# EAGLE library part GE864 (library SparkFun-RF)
Telit quad cell module (see CEL-09296)
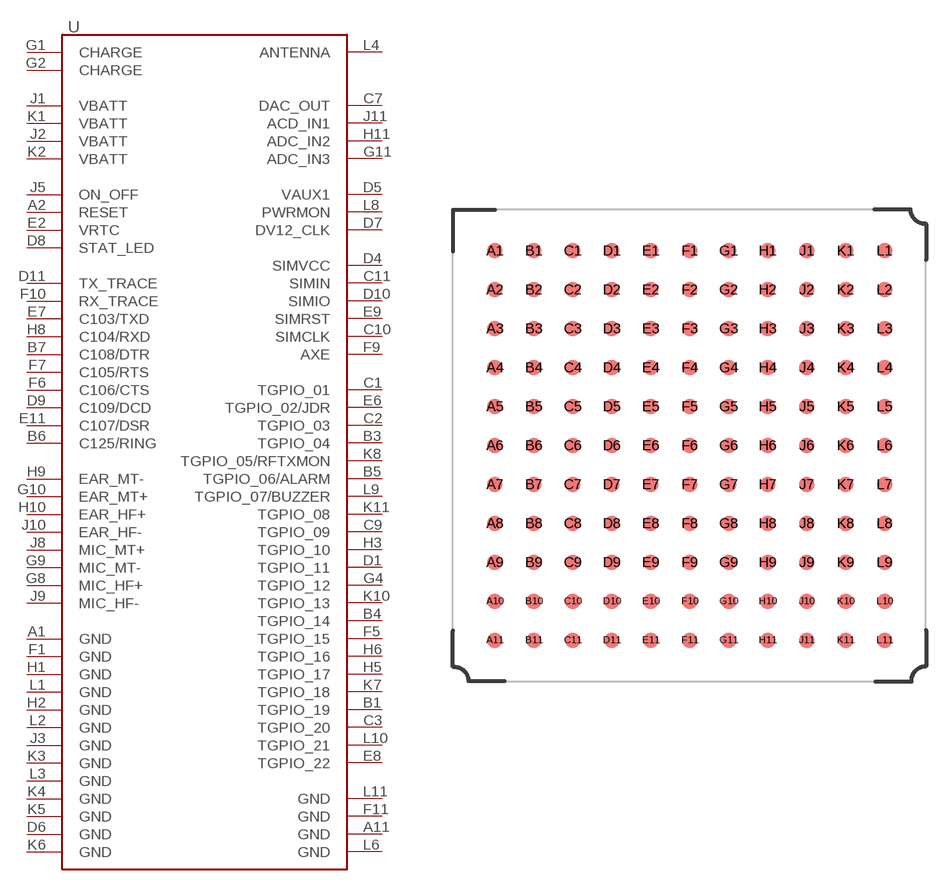
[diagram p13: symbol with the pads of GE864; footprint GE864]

Designator prefix -

## GE864  [GE864]
A1  GND
A2  RESET
A11  GND
B1  TGPIO_19
B3  TGPIO_04
B4  TGPIO_14
B5  TGPIO_06/ALARM
B6  C125/RING
B7  C108/DTR
C1  TGPIO_01
C2  TGPIO_03
C3  TGPIO_20
C7  DAC_OUT
C9  TGPIO_09
C10  SIMCLK
C11  SIMIN
D1  TGPIO_11
D4  SIMVCC
D5  VAUX1
D6  GND
D7  DV12_CLK
D8  STAT_LED
D9  C109/DCD
D10  SIMIO
D11  TX_TRACE
E2  VRTC
E6  TGPIO_02/JDR
E7  C103/TXD
E8  TGPIO_22
E9  SIMRST
E11  C107/DSR
F1  GND
F5  TGPIO_15
F6  C106/CTS
F7  C105/RTS
F9  AXE
F10  RX_TRACE
F11  GND
G1  CHARGE
G2  CHARGE
G4  TGPIO_12
G8  MIC_HF+
G9  MIC_MT-
G10  EAR_MT+
G11  ADC_IN3
H1  GND
H2  GND
H3  TGPIO_10
H5  TGPIO_17
H6  TGPIO_16
H8  C104/RXD
H9  EAR_MT-
H10  EAR_HF+
H11  ADC_IN2
J1  VBATT
J2  VBATT
J3  GND
J5  ON_OFF
J8  MIC_MT+
J9  MIC_HF-
J10  EAR_HF-
J11  ACD_IN1
K1  VBATT
K2  VBATT
K3  GND
K4  GND
K5  GND
K6  GND
K7  TGPIO_18
K8  TGPIO_05/RFTXMON
K10  TGPIO_13
K11  TGPIO_08
L1  GND
L2  GND
L3  GND
L4  ANTENNA
L6  GND
L8  PWRMON
L9  TGPIO_07/BUZZER
L10  TGPIO_21
L11  GND

## Footprint GE864 (pad centres in mm)
smd 1 x 1: A1 0,25; A2 0,22.5; A3 0,20; A4 0,17.5; A5 0,15; A6 0,12.5; A7 0,10; A8 0,7.5; A9 0,5; A10 0,2.5; A11 0,0; B1 2.5,25; B2 2.5,22.5; B3 2.5,20; B4 2.5,17.5; B5 2.5,15; B6 2.5,12.5; B7 2.5,10; B8 2.5,7.5; B9 2.5,5; B10 2.5,2.5; B11 2.5,0; C1 5,25; C2 5,22.5; C3 5,20; C4 5,17.5; C5 5,15; C6 5,12.5; C7 5,10; C8 5,7.5; C9 5,5; C10 5,2.5; C11 5,0; D1 7.5,25; D2 7.5,22.5; D3 7.5,20; D4 7.5,17.5; D5 7.5,15; D6 7.5,12.5; D7 7.5,10; D8 7.5,7.5; D9 7.5,5; D10 7.5,2.5; D11 7.5,0; E1 10,25; E2 10,22.5; E3 10,20; E4 10,17.5; E5 10,15; E6 10,12.5; E7 10,10; E8 10,7.5; E9 10,5; E10 10,2.5; E11 10,0; F1 12.5,25; F2 12.5,22.5; F3 12.5,20; F4 12.5,17.5; F5 12.5,15; F6 12.5,12.5; F7 12.5,10; F8 12.5,7.5; F9 12.5,5; F10 12.5,2.5; F11 12.5,0; G1 15,25; G2 15,22.5; G3 15,20; G4 15,17.5; G5 15,15; G6 15,12.5; G7 15,10; G8 15,7.5; G9 15,5; G10 15,2.5; G11 15,0; H1 17.5,25; H2 17.5,22.5; H3 17.5,20; H4 17.5,17.5; H5 17.5,15; H6 17.5,12.5; H7 17.5,10; H8 17.5,7.5; H9 17.5,5; H10 17.5,2.5; H11 17.5,0; J1 20,25; J2 20,22.5; J3 20,20; J4 20,17.5; J5 20,15; J6 20,12.5; J7 20,10; J8 20,7.5; J9 20,5; J10 20,2.5; J11 20,0; K1 22.5,25; K2 22.5,22.5; K3 22.5,20; K4 22.5,17.5; K5 22.5,15; K6 22.5,12.5; K7 22.5,10; K8 22.5,7.5; K9 22.5,5; K10 22.5,2.5; K11 22.5,0; L1 25,25; L2 25,22.5; L3 25,20; L4 25,17.5; L5 25,15; L6 25,12.5; L7 25,10; L8 25,7.5; L9 25,5; L10 25,2.5; L11 25,0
